(* 	
	Program Name: 	ACS_MOVE_INCREMENTAL_ROTARY_POSITIVE
	Purpose:		Copy Incremental Move Profile to ACS Drive Output Registers
	When Executed:	Primes Output Registers for an Incremental Rotary Move in the Positive Direction to be executed upon Start Motion command
	Note: 			Behavior differs from Incremental Linear Move, see TMI for further details
*)
PROGRAM ACS_MOVE_INCREMENTAL_ROTARY_POSITIVE
VAR_IN_OUT
	Axis:ACS_DRIVE_TYPE;
END_VAR

VAR_INPUT
	// Distance to move in rotary units
	ProfileDistance		:REAL;
	// Velocity in rotary units
	ProfileVelocity		:REAL;
	// Acceleration in rotary units
	ProfileAcceleration	:REAL;
	//Deceleration in rotary units
	ProfileDeceleration	:REAL;
	// Force as % Peak motor current
	ProfileForce		:REAL;
END_VAR

VAR
	_moveType:UDINT := ACS_MOTION_TYPES.ROTARY_INCREMENTAL_POSITIVE;
	// Target Index
	_moveSelect:USINT := 0;
END_VAR

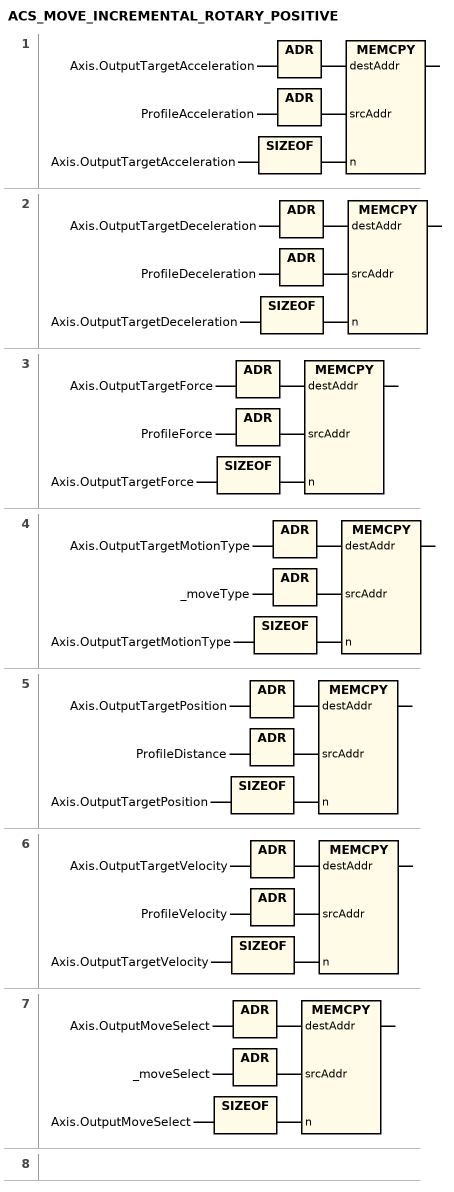
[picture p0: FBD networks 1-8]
// NETWORK 1
MEMCPY(destAddr := ADR(Axis.OutputTargetAcceleration), srcAddr := ADR(ProfileAcceleration), n := SIZEOF(Axis.OutputTargetAcceleration));

// NETWORK 2
MEMCPY(destAddr := ADR(Axis.OutputTargetDeceleration), srcAddr := ADR(ProfileDeceleration), n := SIZEOF(Axis.OutputTargetDeceleration));

// NETWORK 3
MEMCPY(destAddr := ADR(Axis.OutputTargetForce), srcAddr := ADR(ProfileForce), n := SIZEOF(Axis.OutputTargetForce));

// NETWORK 4
MEMCPY(destAddr := ADR(Axis.OutputTargetMotionType), srcAddr := ADR(_moveType), n := SIZEOF(Axis.OutputTargetMotionType));

// NETWORK 5
MEMCPY(destAddr := ADR(Axis.OutputTargetPosition), srcAddr := ADR(ProfileDistance), n := SIZEOF(Axis.OutputTargetPosition));

// NETWORK 6
MEMCPY(destAddr := ADR(Axis.OutputTargetVelocity), srcAddr := ADR(ProfileVelocity), n := SIZEOF(Axis.OutputTargetVelocity));

// NETWORK 7
MEMCPY(destAddr := ADR(Axis.OutputMoveSelect), srcAddr := ADR(_moveSelect), n := SIZEOF(Axis.OutputMoveSelect));

// NETWORK 8

END_PROGRAM
